ORGANIZATION_BLOCK MAIN:OB1
TITLE=

BEGIN
NETWORK 1
LD Q0.0
A I0.2
O I0.1
A I0.0
= S0.0

NETWORK 2
LSCR S0.0

NETWORK 3
LD I0.0
= Q0.0

NETWORK 4
LD Q0.1
ON Q0.2
TON T32 +50

NETWORK 5
LDN T32
AN Q0.2
= Q0.1

NETWORK 6
LD T32
O Q0.2
AN Q0.1
= Q0.2

NETWORK 7
SCRE

NETWORK 8
LDN Q0.0
= Q0.3

NETWORK 9
LD Q0.1
= Q0.4

NETWORK 10
LD Q0.2
= Q0.5

END_ORGANIZATION_BLOCK

